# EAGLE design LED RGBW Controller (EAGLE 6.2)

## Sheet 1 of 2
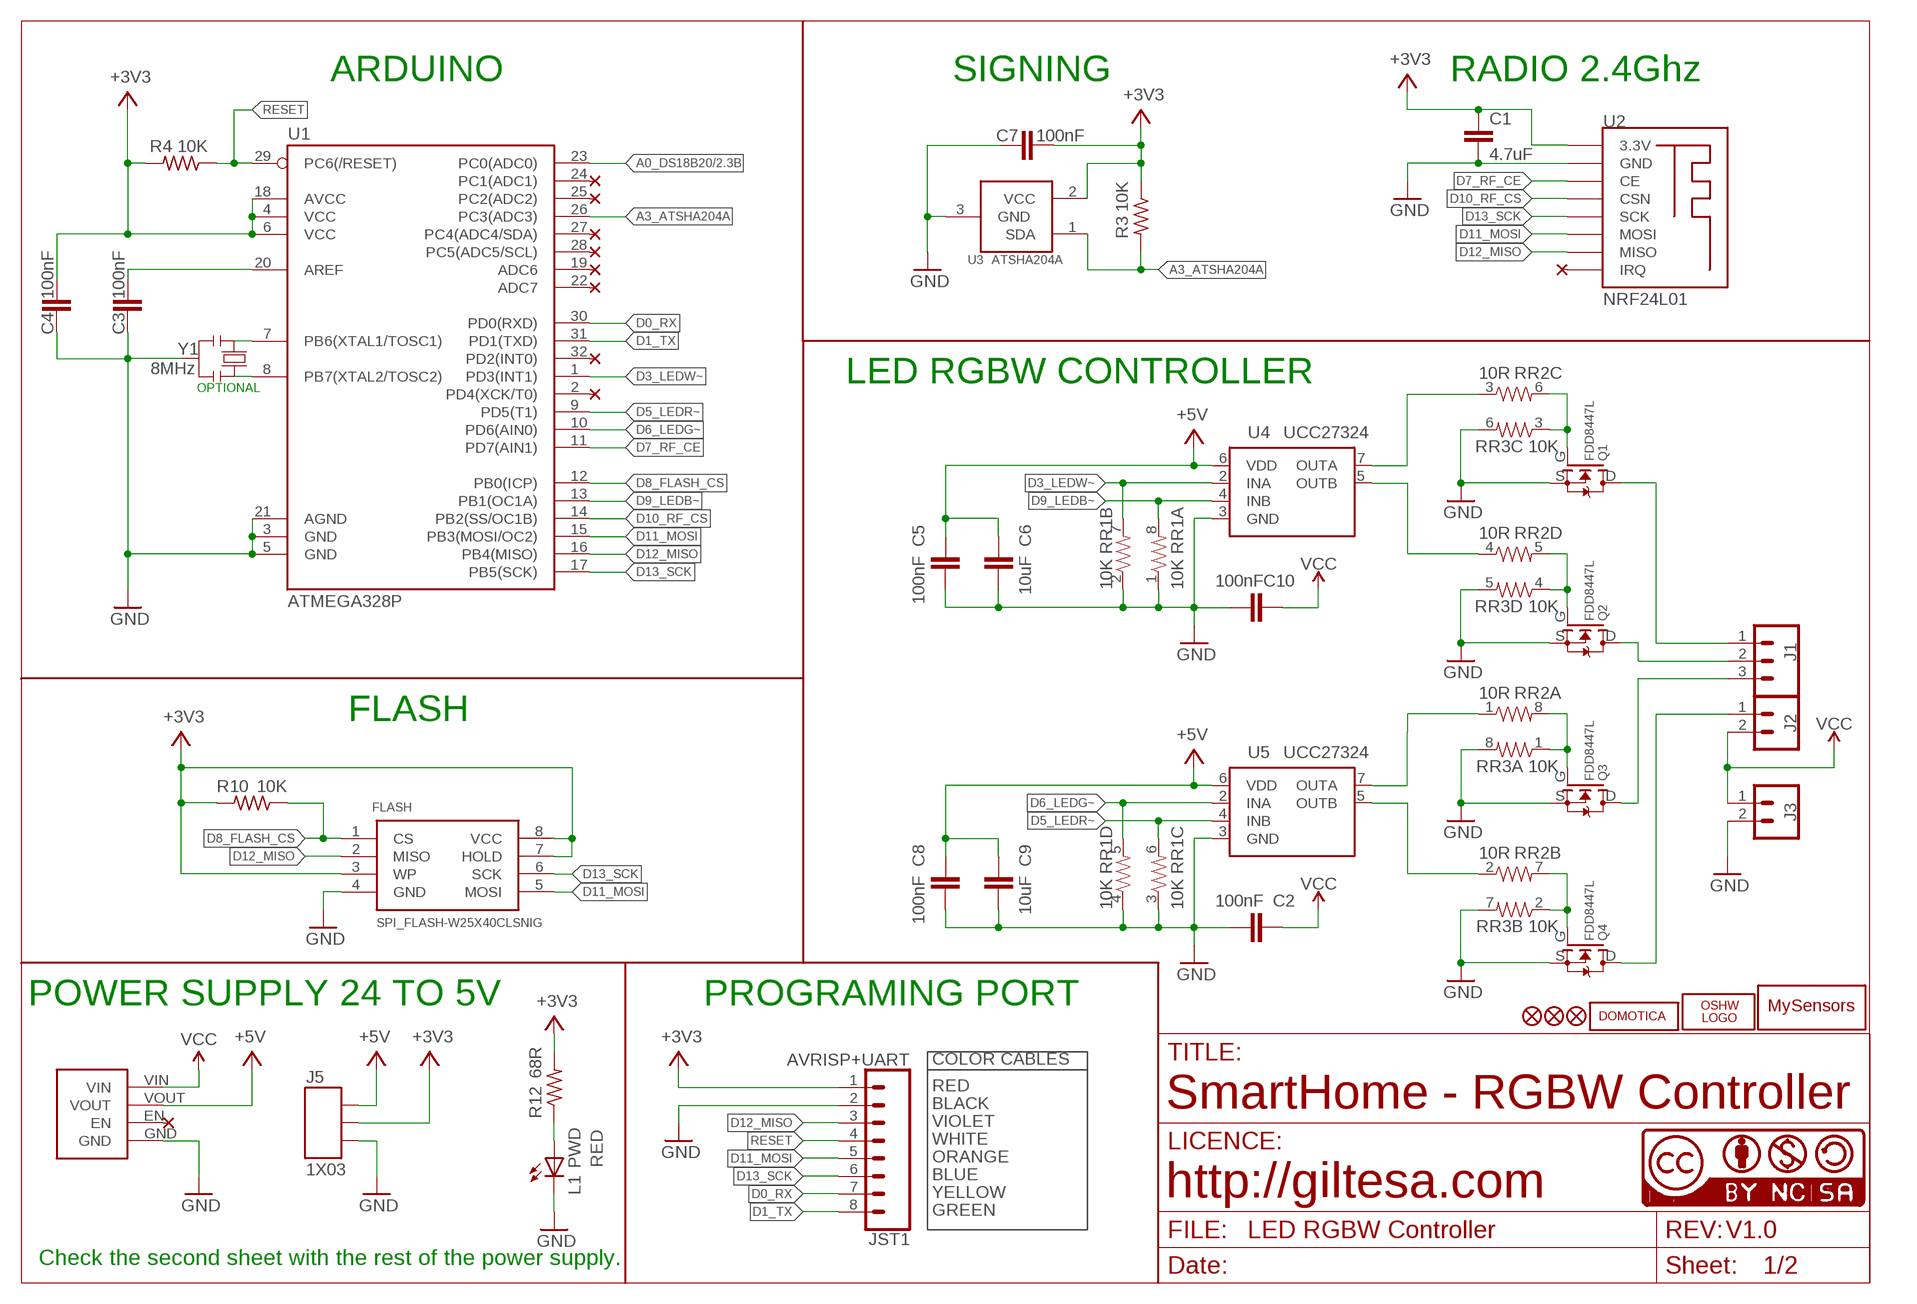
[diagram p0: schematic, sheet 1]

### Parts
C1  4.7uF  C1206  [C1206]
C2  100nF  C0603  [C0603]
C3  100nF  C0603  [C0603]
C4  100nF  C0603  [C0603]
C5  100nF  C0603  [C0603]
C6  10uF  C0603  [C0603]
C7  100nF  C0603  [C0603]
C8  100nF  C0603  [C0603]
C9  10uF  C0603  [C0603]
C10  100nF  C0603  [C0603]
FLASH  SPI_FLASH-W25X40CLSNIG  SPI_FLASH-X25XXSMD  [SO08]
J1  TERMINAL_5MM_3P  [TERMINAL_5MM_3P]
J2  TERMINAL_5MM_2P1  [TERMINAL_5MM_2P]
J3  TERMINAL_5MM_2P1  [TERMINAL_5MM_2P]
J4  DC_CONVERTER  [DC_CONVERTER]
J5  1X03  [1X03_SMD]
JST1  AVRISP+UART  JST-8-1MM-SMD1  [JST-8-1MM-SMD]
L1  PWD  LEDCHIP-LED0805  [CHIP-LED0805]
LOGO1  OSHW_LOGO_FILLX0150-NT  [OSHW_FILLX150_NOTEXT]
Q1  FDD8447L  [TO-252]
Q2  FDD8447L  [TO-252]
Q3  FDD8447L  [TO-252]
Q4  FDD8447L  [TO-252]
R3  10K  R0603  [R0603]
R4  10K  R0603  [R0603]
R10  10K  R0603  [R0603]
R12  68R  R0603  [R0603]
RR1  10K  RESISTOR-ARRAY0603-ARV  [0603-ARV]
RR2  10R  RESISTOR-ARRAY0603-ARV  [0603-ARV]
RR3  10K  RESISTOR-ARRAY0603-ARV  [0603-ARV]
U1  ATMEGA328P  ATMEGA328P_TQFP  [TQFP32-08]
U2  NRF24L01  NRF24L01_SMD  [NRF24L01_SMD]
U3  ATSHA204A  IC_ATSHA204A_CRYPT  [SOT23-3]
U4  UCC27324  [SO8]
U5  UCC27324  [SO8]
U$2  MYSENSORS3  [MYSENSORS_15MM]
U$5  DOMOTICA10MM_2  [DOMOTICA-10MM_2]
U$6  FIDUCIAL1X2  [FIDUCIAL-1X2]
U$7  FIDUCIAL1X2  [FIDUCIAL-1X2]
U$12  CC-BY-NC-SA15MM  [CC-BY-NC-SA_15MM]
U$14  FIDUCIAL1X2  [FIDUCIAL-1X2]
U$18  CC-NC-BCNIX  [CC-NC-B_NIX]
Y1  8MHz  RESONATORMU  [RESONATOR]

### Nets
+3V3: C1.1 C4.2 C7.2 FLASH.3(WP) FLASH.7(HOLD) FLASH.8(VCC) J5.2 JST1.1 R3.1 R4.2 R10.2 R12.2 U1.4(VCC) U1.6(VCC) U1.18(AVCC) U2.3.3V U3.2(VCC) ; also sheet 2
+5V: C5.2 C6.2 C8.2 C9.2 J4.VOUT J5.3 U4.6(VDD) U5.6(VDD)
A0_DS18B20: U1.23(PC0(ADC0)) ; also sheet 2
A3_ATSHA204A: R3.2 U1.26(PC3(ADC3)) U3.1(SDA)
D0_RX: JST1.7 U1.30(PD0(RXD))
D1_TX: JST1.8 U1.31(PD1(TXD))
D3_LEDW~: RR1.7 U1.1(PD3(INT1)) U4.2(INA)
D5_LEDR~: RR1.6 U1.9(PD5(T1)) U5.4(INB)
D6_LEDG~: RR1.5 U1.10(PD6(AIN0)) U5.2(INA)
D7_RF_CE: U1.11(PD7(AIN1)) U2.CE
D8_FLASH_CS: FLASH.1(CS) R10.1 U1.12(PB0(ICP))
D9_LEDB~: RR1.8 U1.13(PB1(OC1A)) U4.4(INB)
D10_RF_CS: U1.14(PB2(SS/OC1B)) U2.CSN
D11_MOSI: FLASH.5(MOSI) JST1.5 U1.15(PB3(MOSI/OC2)) U2.MOSI
D12_MISO: FLASH.2(MISO) JST1.3 U1.16(PB4(MISO)) U2.MISO
D13_SCK: FLASH.6(SCK) JST1.6 U1.17(PB5(SCK)) U2.SCK
GND: C1.2 C2.1 C3.1 C4.1 C5.1 C6.1 C7.1 C8.1 C9.1 C10.1 FLASH.4(GND) J3.2 J4.GND J5.1 JST1.2 L1.C Q1.S Q2.S Q3.S Q4.S RR1.1 RR1.2 RR1.3 RR1.4 RR3.5 RR3.6 RR3.7 RR3.8 U1.3(GND) U1.5(GND) U1.21(AGND) U2.GND U3.3(GND) U4.3(GND) U5.3(GND) Y1.2 ; also sheet 2
N$1: J1.1 Q1.D
N$2: Q2.G RR2.5 RR3.4
N$3: J1.2 Q2.D
N$4: Q3.G RR2.8 RR3.1
N$5: J1.3 Q3.D
N$6: Q1.G RR2.6 RR3.3
N$7: Q4.G RR2.7 RR3.2
N$8: J2.1 Q4.D
N$9: L1.A R12.1
N$10: RR2.3 U4.7(OUTA)
N$11: RR2.4 U4.5(OUTB)
N$12: RR2.1 U5.7(OUTA)
N$13: RR2.2 U5.5(OUTB)
N$29: U1.7(PB6(XTAL1/TOSC1)) Y1.1
N$30: U1.8(PB7(XTAL2/TOSC2)) Y1.3
N$33: C3.2 U1.20(AREF)
RESET: JST1.4 R4.1 U1.29(PC6(/RESET))
VCC: C2.2 C10.2 J2.2 J3.1 J4.VIN
Unconnected: J4.EN U1.2(PD4(XCK/T0)) U1.19(ADC6) U1.22(ADC7) U1.24(PC1(ADC1)) U1.25(PC2(ADC2)) U1.27(PC4(ADC4/SDA)) U1.28(PC5(ADC5/SCL)) U1.32(PD2(INT0)) U2.IRQ

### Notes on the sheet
- ARDUINO | SIGNING | RADIO 2.4Ghz
- LED RGBW CONTROLLER
- OPTIONAL
- FLASH
- POWER SUPPLY 24 TO 5V | PROGRAMING PORT
- COLOR CABLES
- RED
- BLACK | SmartHome - RGBW Controller
- VIOLET
- WHITE
- RED | ORANGE
- BLUE
- YELLOW | http://giltesa.com
- GREEN
- V1.0
- Check the second sheet with the rest of the power supply.

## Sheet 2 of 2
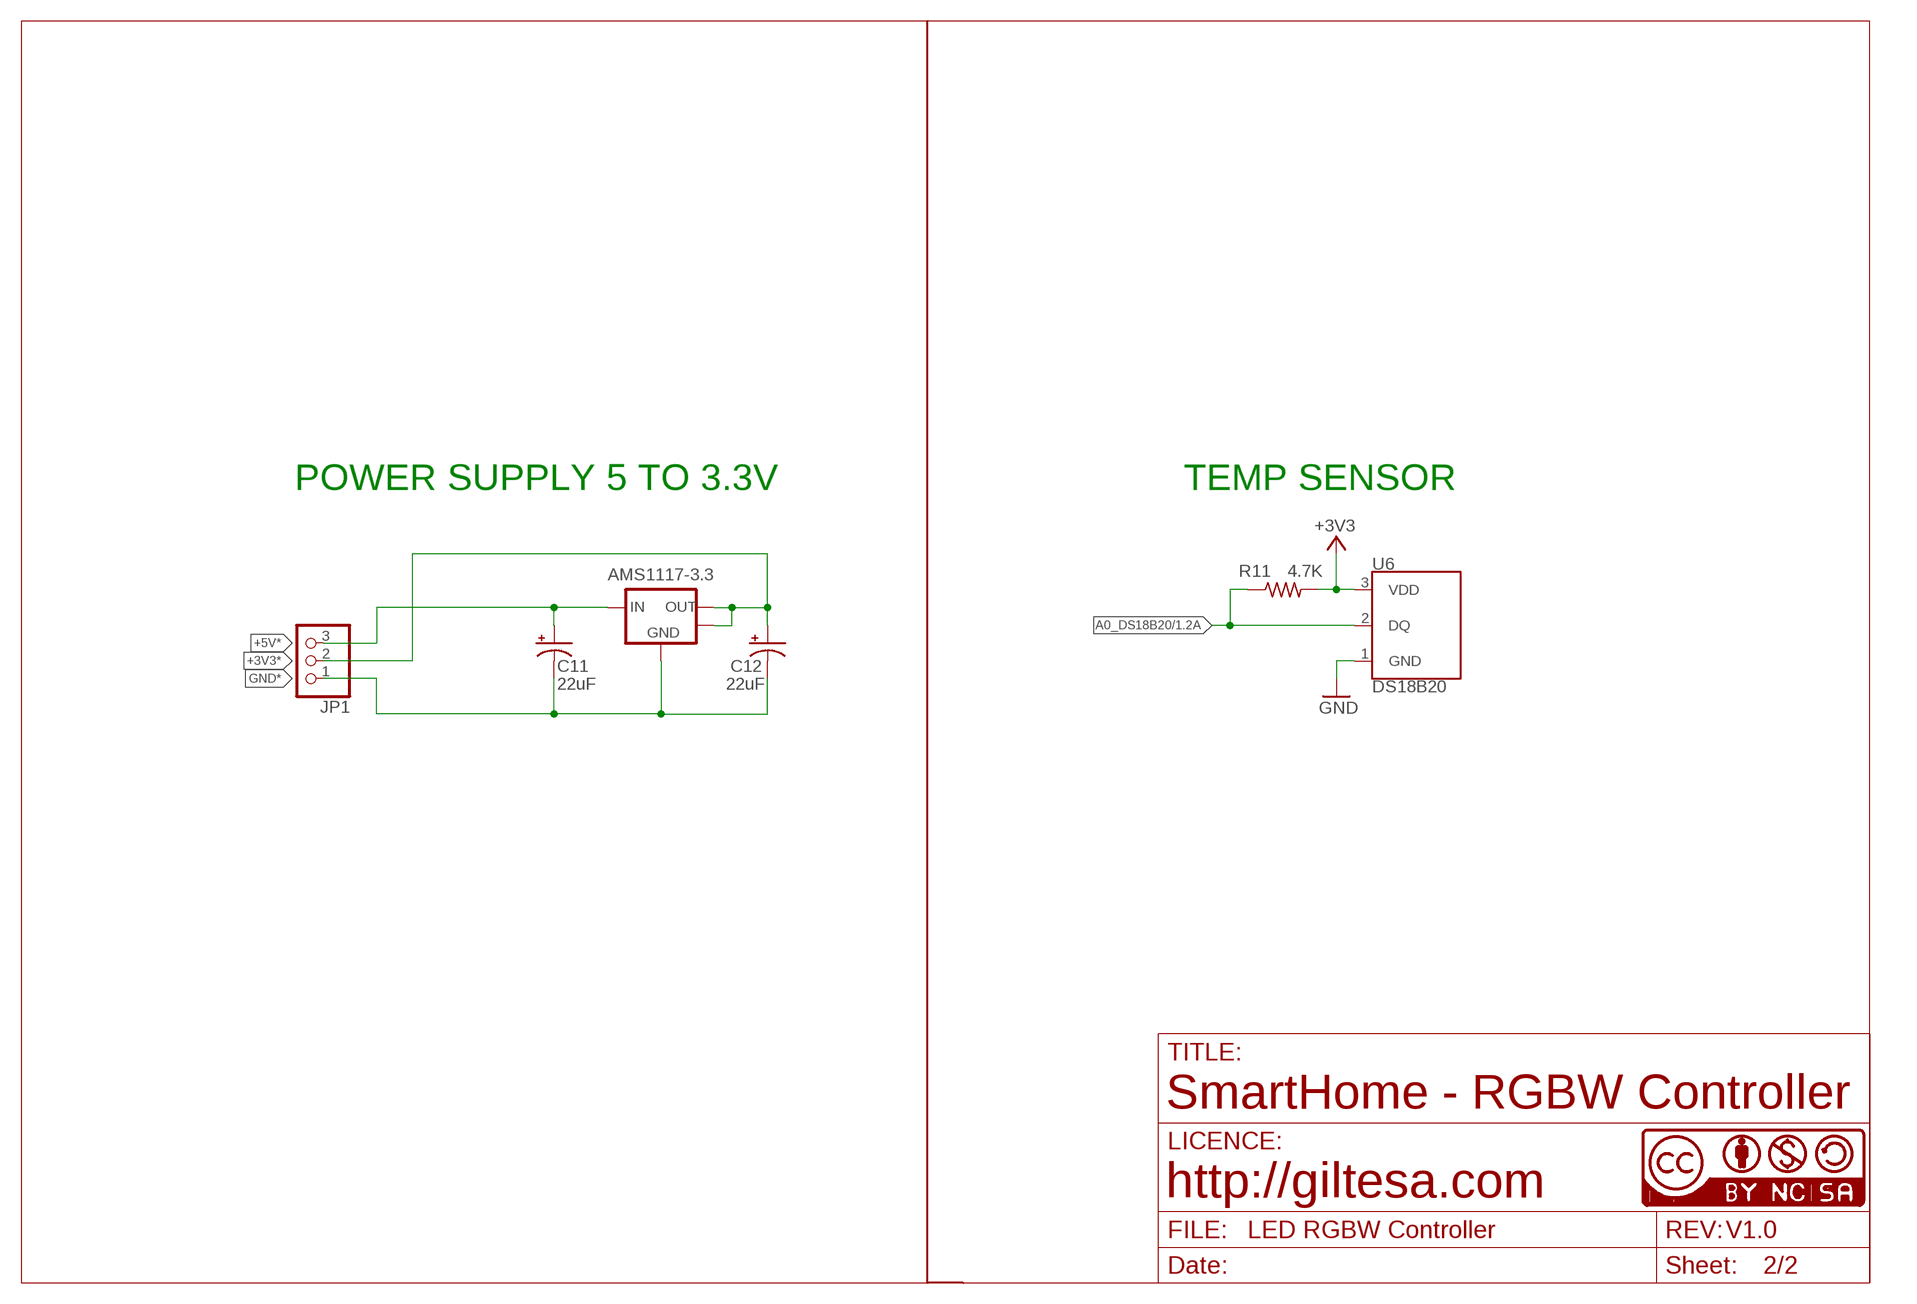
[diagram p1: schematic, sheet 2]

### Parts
AMS1117-3.3  AMS1117-3.3  AMS1117SOT89_2  [SOT89_2]
C11  22uF  CAP_POL3528  [EIA3528]
C12  22uF  CAP_POL3528  [EIA3528]
JP1  PINHD-1X3  [1X03]
R11  4.7K  R0603  [R0603]
U6  DS18B20  [DS18B20]
U$21  CC-NC-BCNIX  [CC-NC-B_NIX]

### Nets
+3V3: R11.2 U6.3(VDD) ; also sheet 1
+3V3*: AMS1117-3.3.2(OUT) AMS1117-3.3.4(NC) C12.A(+) JP1.2
+5V*: AMS1117-3.3.3(IN) C11.A(+) JP1.3
A0_DS18B20: R11.1 U6.2(DQ) ; also sheet 1
GND: U6.1(GND) ; also sheet 1
GND*: AMS1117-3.3.1(GND) C11.C(-) C12.C(-) JP1.1

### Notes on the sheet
- POWER SUPPLY 5 TO 3.3V | TEMP SENSOR
- SmartHome - RGBW Controller
- http://giltesa.com
- V1.0

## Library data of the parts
AMS1117-3.3 = ,giltesa:AMS1117
C1 = ,giltesa:C1206
C2-C10 = ,giltesa:C0603
C11 C12 = SparkFun:CAP_POL: Capacitor Polarized
FLASH = SparkFun-DigitalIC:SPI_FLASH-X25XX: 8pin SPI Flash series x25xx. Works with devices like W25X32 and BR25L32
J1 = ,giltesa:TERMINAL_5MM_3P
J2 J3 = ,giltesa:TERMINAL_5MM_2P
J4 = ,giltesa:DC_CONVERTER
J5 = ,giltesa:1X03
JP1 = adafruit:PINHD-1X3: PIN HEADER
JST1 = ,giltesa:JST-8-1MM-SMD
L1 = led:LED: LED
LOGO1 = ohw-logo:OSHW_LOGO_FILL
Q1-Q4 = ,giltesa:FDD8447L
R3 R4 R10-R12 = ,giltesa:R0603
RR1-RR3 = SparkFun-Passives:RESISTOR-ARRAY: Array Chip Resistor Source: RS Component / Phycomp
U1 = SparkFun-DigitalIC:ATMEGA328P_TQFP; PROD_ID: IC-09069; VALUE: ATMEGA328P_TQFP
U2 = ,giltesa:NRF24L01_SMD
U3 = TD-MySensors:IC_ATSHA204A_CRYPT
U4 U5 = ,giltesa:UCC27324
U6 = ,giltesa:DS18B20
U$2 = ,giltesa_logos:MYSENSORS
U$5 = ,giltesa_logos:DOMOTICA
U$6 U$7 U$14 = SparkFun:FIDUCIAL: Fiducial Alignment Points
U$12 = ,giltesa_logos:CC-BY-NC-SA
U$18 U$21 = cc-by-nc-sa:CC-NC-BC: All hardware is licensed under the Creative Commons
Y1 = MySMD2:RESONATOR

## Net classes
2 gnd: width 0.305 mm, drill 0.406 mm, clearance 0.203 mm
3 usbvcc: width 0.203 mm, drill 0.406 mm, clearance 0.203 mm
4 USBpair: width 0.254 mm, drill 0.406 mm, clearance 0.61 mm

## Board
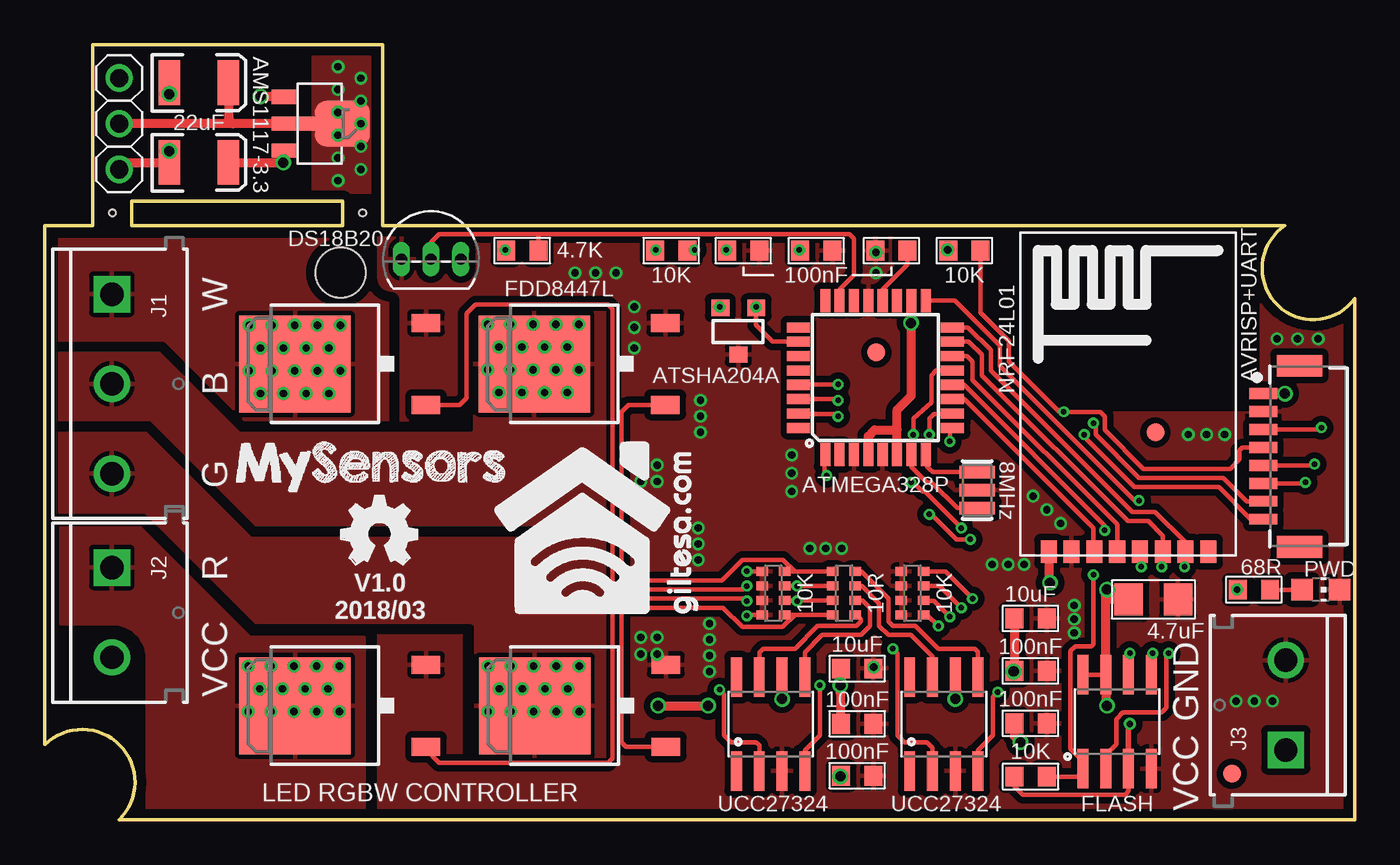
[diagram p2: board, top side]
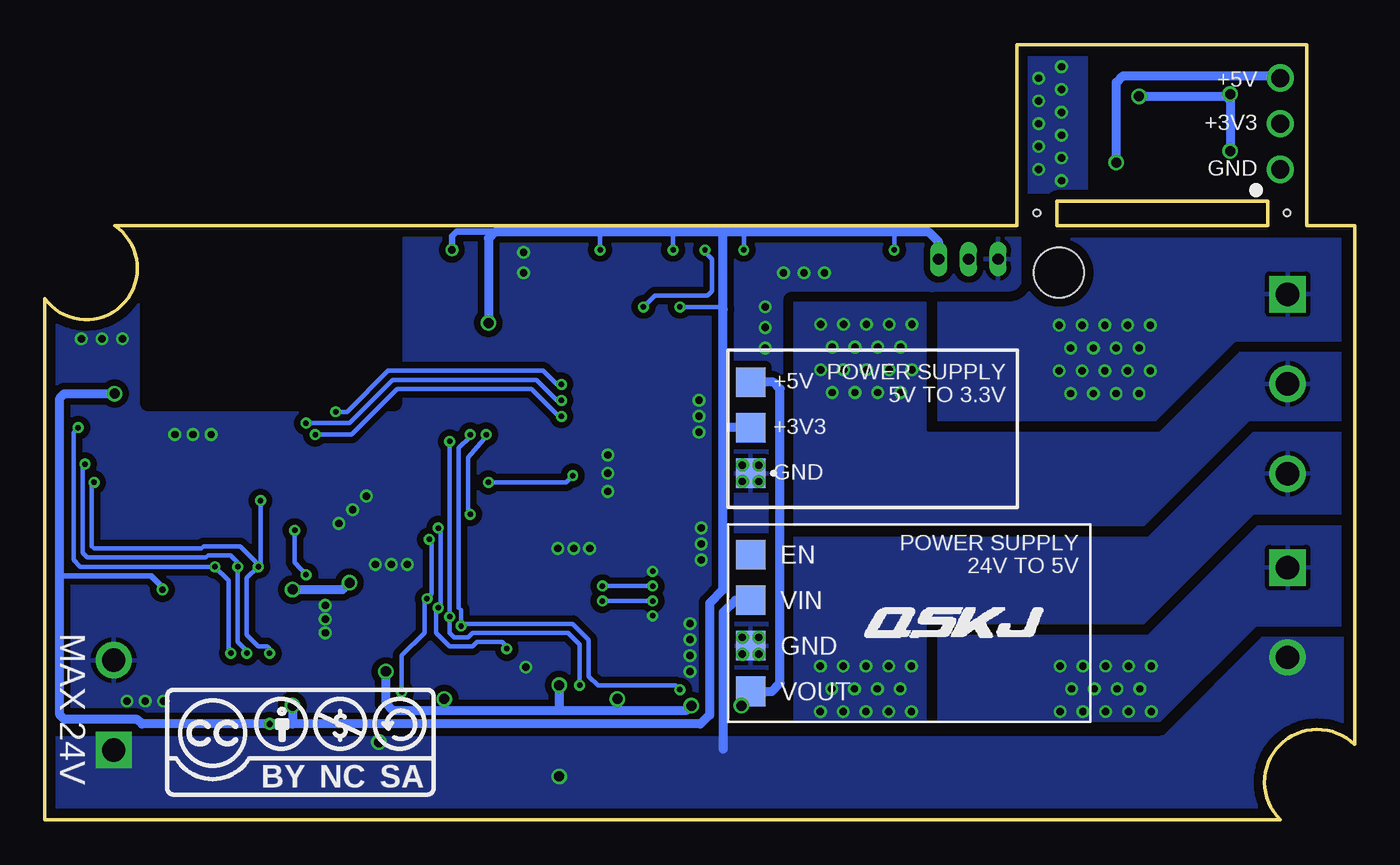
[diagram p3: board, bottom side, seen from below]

Size 72.97 x 43.18 mm. Coordinates in mm from the lower left corner, seen from the top.
Outline: 4.14,0 72.97,0 72.97,29.03 arc-200 69.09,33.1 18.82,33.1 18.82,43.18 2.67,43.18 2.67,33.1 0,33.1 0,4.19 0.03,4.19 arc-180 4.14,0
Outline: 16.59,33.1 4.85,33.1 4.85,34.47 16.59,34.47 16.59,33.1
Copper layers (1*16): Top 0.035mm / dielectric 1.6mm / Bottom 0.035mm
Design rules: minimum track width 6mil, minimum drill 12mil, track to track 6mil, track to pad 6mil, pad to pad 6mil, via to via 8mil, smd to smd 0mil, copper to edge 20mil, drill to drill 10mil, minimum pad ring 6mil, minimum via ring 6mil, stop-mask expansion 0mil, vias tented up to drill 100mil, thermal gap 10mil
Holes 0.38 mm at 17.7,33.81 3.76,33.81
Holes 2.79 mm at 16.47,30.49
tRestrict: 41 lines
bRestrict: 44 lines

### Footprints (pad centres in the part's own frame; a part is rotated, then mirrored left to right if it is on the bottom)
SOT89_2 = smd 0.8 x 1.4: 1 -1.499,-1.981; 3 1.499,-1.981 | smd 0.8 x 2.54: 2 0,-1.409 | smd 2.54 x 3.048: 4 0,1.27
C1206 = smd 1.6 x 1.8: 1 -1.362,-0.013; 2 1.387,-0.013
C0603 = smd 1 x 1.1: 1 -0.901,-0.038; 2 0.901,-0.038
EIA3528 = smd 1.2 x 2.5: A 1.65,0; C -1.65,0
SO08 = smd 0.61 x 2.21: 1 -1.905,-2.616; 2 -0.635,-2.616; 3 0.635,-2.616; 4 1.905,-2.616; 5 1.905,2.616; 6 0.635,2.616; 7 -0.635,2.616; 8 -1.905,2.616
TERMINAL_5MM_3P = drill 1.3 pad 2.032 square: 1 0,0 | drill 1.3 pad 2.032: 2 5,0; 3 10,0
TERMINAL_5MM_2P = drill 1.3 pad 2.032 square: 1 0,0 | drill 1.3 pad 2.032: 2 5,0
DC_CONVERTER = smd 1.651 x 1.651: EN 1.27,9.31; GND 1.27,4.23; VIN 1.27,6.77; VOUT 1.27,1.69
1X03_SMD = smd 1.651 x 1.651: 1 0,-2.54; 2 0,0; 3 0,2.54
1X03 = drill 1.016: 1 -2.54,0; 2 0,0; 3 2.54,0
JST-8-1MM-SMD = smd 0.6 x 1.55: 1 -3.5,-2.017; 2 -2.5,-2.017; 3 -1.5,-2.017; 4 -0.5,-2.017; 5 0.5,-2.017; 6 1.5,-2.017; 7 2.5,-2.017; 8 3.5,-2.017 | smd 1.219 x 2.54: NC1 -5.054,0; NC2 5.054,0
CHIP-LED0805 = smd 1.2 x 1.2: A 0,-1.05; C 0,1.05
TO-252 = smd 5.4 x 6.2: D 0,2.5 | smd 1 x 1.6: G -2.28,-4.8; S 2.28,-4.8
R0603 = smd 1 x 1.1: 1 -0.901,0.013; 2 0.901,0.013
0603-ARV = smd 0.5 x 0.65: 1 -1.2,-0.625; 2 -0.4,-0.625; 3 0.4,-0.625; 4 1.2,-0.625; 5 1.2,0.625; 6 0.4,0.625; 7 -0.4,0.625; 8 -1.2,0.625
TQFP32-08 = smd 1.27 x 0.559: 1 -4.293,2.8; 2 -4.293,2; 3 -4.293,1.2; 4 -4.293,0.4; 5 -4.293,-0.4; 6 -4.293,-1.2; 7 -4.293,-2; 8 -4.293,-2.8; 17 4.293,-2.8; 18 4.293,-2; 19 4.293,-1.2; 20 4.293,-0.4; 21 4.293,0.4; 22 4.293,1.2; 23 4.293,2; 24 4.293,2.8 | smd 0.559 x 1.27: 9 -2.8,-4.293; 10 -2,-4.293; 11 -1.2,-4.293; 12 -0.4,-4.293; 13 0.4,-4.293; 14 1.2,-4.293; 15 2,-4.293; 16 2.8,-4.293; 25 2.8,4.293; 26 2,4.293; 27 1.2,4.293; 28 0.4,4.293; 29 -0.4,4.293; 30 -1.2,4.293; 31 -2,4.293; 32 -2.8,4.293
NRF24L01_SMD = smd 0.9 x 1.27: 3.3V 1.575,0.203; CE 4.115,0.203; CSN 5.385,0.203; GND 2.845,0.203; IRQ 10.465,0.203; MISO 9.195,0.203; MOSI 7.925,0.203; SCK 6.655,0.203
SOT23-3 = smd 1 x 0.9: 1 -1,-1.3; 2 1,-1.3; 3 0,1.3
SO8 = smd 0.61 x 2.21: 1 -1.905,-2.616; 2 -0.635,-2.616; 3 0.635,-2.616; 4 1.905,-2.616; 5 1.905,2.616; 6 0.635,2.616; 7 -0.635,2.616; 8 -1.905,2.616
DS18B20 = drill 0.635 pad 0.864 long: 1 -1.651,0; 2 0,0; 3 1.651,0
FIDUCIAL-1X2 = smd 1 x 1: 1 0,0
RESONATOR = smd 0.7 x 2: 1 -1,0; 2 0,0; 3 1,0

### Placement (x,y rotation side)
AMS1117-3.3  15.32,38.79 270 top
C1  61.75,12.29 0 top
C2  45.26,2.41 180 top
C3  47.17,31.75 0 top
C4  42.98,31.67 180 top
C5  54.91,8.26 180 top
C6  54.91,11.18 180 top
C7  38.91,31.67 180 top
C8  45.26,5.31 180 top
C9  45.26,8.38 180 top
C10  54.91,5.33 180 top
C11  8.59,36.63 0 top
C12  8.59,41.07 0 top
FLASH  59.74,5.46 0 top
J1  3.73,29.29 270 top
J2  3.73,14.05 270 top
J3  69.14,3.89 90 top
J4  34.92,5.46 0 bottom
J5  33.66,21.84 0 bottom
JP1  4.14,38.79 90 top
JST1  69.9,20.24 270 top
L1  71.09,12.83 270 top
LOGO1  16.51,14.22 0 top
Q1  16.43,25.4 90 top
Q2  29.77,25.4 90 top
Q3  29.79,6.35 90 top
Q4  16.43,6.35 90 top
R3  34.9,31.7 0 top
R4  51.23,31.72 180 top
R10  54.91,2.41 180 top
R11  26.59,31.72 180 top
R12  67.36,12.83 180 top
RR1  48.34,12.62 270 top
RR2  44.53,12.62 90 top
RR3  40.59,12.62 90 top
U1  46.28,24.64 90 top
U2  54.36,14.73 0 top
U3  38.63,27.23 180 top
U4  50.09,5.33 0 top
U5  40.44,5.33 0 top
U6  21.51,31.24 0 top
U$2  10.67,18.29 0 top
U$5  25.65,11.3 0 top
U$6  46.33,26.04 180 top
U$7  61.87,21.59 180 top
U$12  66.29,1.27 0 bottom
U$14  66.14,2.57 180 top
U$18  0,0 180 top
U$21  0,0 180 top
Y1  51.94,18.36 90 top

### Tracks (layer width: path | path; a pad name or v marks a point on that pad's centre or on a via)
+3V3  (via drill 0.3, 0.36, 0.41, 0.56)
  Top 0.254: C4.2 42.08,32.09 v42.04,31.75 | R11.2 25.69,31.96 v25.65,31.75 | C7.2 38.01,31.96 v37.97,31.75 | U3.2 37.38,28.53 v37.59,28.57 | FLASH.8 FLASH.7 | v34.04,31.75 34.01,31.75 R3.1 | R10.2 54.01,1.87 54.48,1.4 60.2,1.4 60.38,1.57 FLASH.3
  Top 0.305: FLASH.3 60.38,5.26 v60.45,5.33 | R12.2 66.53,12.81 v66.42,12.83
  Top 0.356: R4.2 50.33,31.96 v50.29,31.75
  Top 0.508: v69.09,23.75 JST1.1 | v59.18,6.35 59.11,6.43 FLASH.7 59.11,12.32 | 59.11,12.32 59.11,12.88 v59.18,12.83 | 56.01,13.08 v56.01,13.21 55.93,13.28 U2.3.3V | C1.1 59.14,12.28 59.11,12.32 | U1.6 47.48,21.72 | 47.48,21.72 47.48,22.84 48.26,23.62 v48.26,27.69 48.26,28.91 U1.18 | U1.4 45.88,21.37 46.23,21.72 47.48,21.72
  Bottom 0.254: 35.81,32.64 35.69,32.77 | v42.04,31.75 42.04,32.64 41.91,32.77 | v25.65,31.75 25.65,32.77 | v37.97,31.75 37.97,32.64 38.1,32.77 | v37.59,28.57 35.31,28.57 35.18,28.45 | v34.04,31.75 34.04,32.64 34.16,32.77
  Bottom 0.305: v60.45,5.33 60.2,5.33 | v66.42,12.83 66.42,12.95 67.06,13.59 72.14,13.59
  Bottom 0.356: v50.29,31.75 50.29,32.51 50.04,32.77 47.75,32.77
  Bottom 0.508: 59.18,5.33 36.45,5.33 35.94,5.84 35.94,12.06 35.18,12.83 35.18,21.72 | 59.18,5.33 60.2,5.33 67.56,5.33 67.82,5.59 71.88,5.59 72.14,5.84 72.14,13.59 72.14,23.5 71.88,23.75 v69.09,23.75 | 35.18,21.72 35.18,28.45 35.18,32.77 | 35.18,32.77 35.69,32.77 38.1,32.77 41.91,32.77 47.75,32.77 47.88,32.77 48.26,32.38 v48.26,27.69 | 35.18,32.77 34.16,32.77 25.65,32.77 23.75,32.77 23.16,32.18 U6.3 | J5.2 35.05,21.84 35.18,21.72 | v59.18,6.35 59.18,5.33 | v59.18,12.83 56.39,12.83 v56.01,13.21
+3V3*  (via drill 0.41)
  Top 0.508: AMS1117-3.3.4 AMS1117-3.3.2 10.49,38.79 | 10.49,38.79 JP1.2 | C12.A 10.23,39.04 10.49,38.79
  other vias: 17.6,38.79 17.6,40.06 17.6,41.33 17.6,37.52 17.6,36.25 16.33,36.88 16.33,38.15 16.33,39.42 16.33,40.69 16.33,41.96 16.33,35.61
  pour Top (no thermals): 14.94,42.72 18.49,42.72 18.49,34.98 14.94,34.98
  pour Bottom (no thermals): 14.94,42.72 18.49,42.72 18.49,34.98 14.94,34.98
+5V  (via drill 0.56)
  Top 0.508: v34.16,6.35 v36.96,6.35 | v53.98,8.26 v53.98,8.25 C5.2 C6.2 | U4.6 v50.72,6.73 | U5.6 v41.07,6.73 | C8.2 44.36,7.28 | 44.36,6.44 v44.32,7.49 44.36,7.28 | C9.2 44.36,7.28
  Bottom 0.508: J5.3 32.38,24.38 32,24 32,7.62 32.47,7.15 J4.VOUT v34.16,6.35 | v53.98,8.26 53.98,6.48 53.59,6.1 50.85,6.1 | 50.85,6.1 44.45,6.1 | 44.45,6.1 41.07,6.1 | 41.07,6.1 37.21,6.1 v36.96,6.35 | v41.07,6.73 41.07,6.1 | v50.72,6.73 50.72,6.22 50.85,6.1 | v44.32,7.49 44.32,6.22 44.45,6.1
+5V*  (via drill 0.56)
  Top 0.508: AMS1117-3.3.3 13.34,36.68 v13.28,36.63 C11.A
  Bottom 0.508: v13.28,36.63 13.28,41.07 12.9,41.45 4.27,41.45 JP1.3
A0_DS18B20
  Top 0.254: U1.23 44.28,29.55 45.09,30.35 45.09,32.38 44.83,32.64 27.43,32.64 | 27.43,32.64 21.97,32.64 21.51,32.18 U6.2 | R11.1 27.5,32.58 27.43,32.64
A3_ATSHA204A  (via drill 0.3)
  Top 0.254: R3.2 36.16,31.71 v36.2,31.75 | U1.26 40.55,26.64 39.62,27.56 39.62,28.52 | 39.62,28.52 U3.1 39.71,28.45 v39.62,28.57 39.62,28.52
  Bottom 0.254: v36.2,31.75 36.2,31.62 35.81,31.24 35.81,29.46 36.07,29.21 38.99,29.21 v39.62,28.57 39.5,28.7
D0_RX  (via drill 0.3)
  Top 0.254: JST1.7 66.97,17.74 65.66,19.05 60.96,19.05 58.55,21.46 58.55,21.97 v58.42,22.1 | U1.30 44.13,23.44 v44.2,23.37
  Bottom 0.254: v44.2,23.37 44.45,23.37 45.59,24.51 53.59,24.51 56.01,22.1 v58.42,22.1
D1_TX  (via drill 0.3)
  Top 0.254: JST1.8 67.2,16.74 65.41,18.54 60.71,18.54 57.91,21.34 v57.91,21.46 | U1.31 42.02,22.61 44.07,22.61 v44.2,22.48
  Bottom 0.254: v44.2,22.48 44.32,22.48 45.85,24 53.34,24 55.88,21.46 v57.91,21.46
D3_LEDW~  (via drill 0.3)
  Top 0.254: U4.2 49.45,4.01 49.15,4.32 47.88,4.32 47.5,4.7 47.5,9.27 v47.24,9.53 | RR1.7 49.84,13.02 v51.05,11.81 | v51.05,16.26 49.02,18.29 48.9,18.29 48.39,18.8 v48.26,18.8 | U1.1 43.43,20.3 43.43,19.3 v43.56,19.18
  Bottom 0.254: v47.24,9.53 47.24,9.65 47.5,9.91 48.9,9.91 49.15,9.65 50.42,9.65 51.18,10.41 51.18,11.68 v51.05,11.81 50.93,11.94 50.93,16.13 v51.05,16.26 | v48.26,18.8 43.94,18.8 v43.56,19.18
D5_LEDR~  (via drill 0.3)
  Top 0.254: RR1.6 48.99,12.19 49.53,12.19 v50.42,11.3 | v43.18,7.49 43.18,4.7 42.34,3.86 U5.4 | v50.42,21.08 50.42,21.69 U1.9
  Bottom 0.254: v43.18,7.49 43.18,9.78 43.81,10.41 49.15,10.41 49.4,10.16 50.16,10.16 50.42,10.41 v50.42,11.3 v50.42,21.08
D6_LEDG~  (via drill 0.3)
  Top 0.254: U5.2 39.8,4.14 39.62,4.32 38.23,4.32 37.85,4.7 37.85,6.99 v37.59,7.24 | RR1.5 49.16,11.42 v49.78,10.79 | v49.28,21.46 49.28,22.35 49.53,22.61 50.54,22.61 U1.10
  Bottom 0.254: v37.59,7.24 37.85,7.49 42.16,7.49 42.67,8 42.67,10.03 43.56,10.92 49.66,10.92 v49.78,10.79 49.78,11.68 49.91,11.81 49.91,20.7 49.28,21.34 v49.28,21.46
D7_RF_CE
  Top 0.254: U2.CE 58.47,15.19 58.42,15.24 58.42,16.26 51.24,23.44 U1.11
D8_FLASH_CS  (via drill 0.3)
  Top 0.254: v58.42,13.65 58.42,9.78 58.29,9.65 57.4,9.65 57.15,9.4 57.15,3.94 57.84,3.25 FLASH.1 57.84,2.41 57.53,2.41 57.52,2.4 R10.1 | U1.12 51.2,24.24 59.05,16.38 v59.05,16.13
  Bottom 0.254: v58.42,13.65 59.05,14.35 v59.05,16.13
D9_LEDB~  (via drill 0.3)
  Top 0.254: U4.4 51.99,3.86 52.83,4.7 52.83,6.86 v53.09,7.11 | RR1.8 48.98,13.84 50.16,13.84 v51.69,12.32 | U1.13 50.55,25.02 49.66,25.02 49.4,24.77 49.4,23.24 48.39,22.35 v48.39,21.46 | v51.56,15.62 50.8,15.62 49.4,17.02 v49.28,17.02
  Bottom 0.254: v53.09,7.11 53.09,9.14 51.82,10.41 51.82,12.19 v51.69,12.32 51.44,12.57 51.44,15.49 v51.56,15.62 | v49.28,17.02 49.4,17.02 49.4,20.19 48.51,21.21 v48.39,21.46
D10_RF_CS
  Top 0.254: U2.CSN 59.74,16.46 51.69,24.51 51.69,25.53 51.38,25.84 U1.14
D11_MOSI  (via drill 0.3)
  Top 0.254: v62.23,14.1 62.28,14.15 U2.MOSI 62.28,15.82 61.47,16.64 60.33,16.64 52.2,24.77 52.2,25.91 51.47,26.64 U1.15 | v61.72,9.27 61.72,8.15 FLASH.5 | JST1.5 70.67,19.74 v70.74,19.81
  Bottom 0.254: v61.72,9.27 61.72,9.4 62.23,9.91 v62.23,14.1 62.23,14.35 62.61,14.73 63.88,14.73 64.01,14.61 70.61,14.61 70.87,14.86 70.87,19.68 v70.74,19.81
D12_MISO  (via drill 0.3)
  Top 0.254: v62.61,9.27 62.48,9.14 62.48,6.22 62.23,5.97 60.07,5.97 59.69,5.59 59.69,4.19 59.11,3.61 FLASH.2 | v63.5,14.1 63.5,14.76 U2.MISO 63.5,14.99 63.5,15.49 61.85,17.14 60.58,17.14 52.7,25.02 52.7,26.16 51.43,27.44 U1.16 | JST1.3 71.02,21.74 v71.12,21.84
  Bottom 0.254: v62.61,9.27 62.74,9.4 62.74,13.34 v63.5,14.1 70.99,14.1 71.37,14.48 71.37,21.59 v71.12,21.84
D13_SCK  (via drill 0.3)
  Top 0.254: U2.SCK 61.01,14.17 v61.09,14.1 | v60.45,9.27 60.45,8.15 FLASH.6 | JST1.6 70.18,18.74 v70.23,18.8 | U1.17 50.7,28.93 53.21,26.42 53.21,25.27 60.83,17.65 v60.96,17.78
  Bottom 0.254: v60.45,9.27 60.45,9.53 60.58,9.65 61.09,9.65 61.72,10.29 61.72,13.46 v61.09,14.1 | v61.09,14.1 61.09,14.22 62.1,15.24 64.14,15.24 64.26,15.11 70.23,15.11 70.36,15.24 70.36,18.67 v70.23,18.8 | v60.96,17.78 60.96,14.22 v61.09,14.1
GND  (via drill 0.3, 0.41)
  Top 0.254: RR3.5 39.13,13.82 v39.12,13.84 | RR3.8 39.12,11.42 v39.12,11.37
  other vias: 33.2,10.16 34.11,10.16 33.2,9.22 34.11,9.22 33.2,18.85 34.11,18.85 33.2,19.76 34.11,19.76 37.03,10.92 37.03,10.03 37.03,9.14 37.03,8.26 65.74,21.46 64.72,21.46 63.7,21.46 68.66,26.8 69.8,26.8 70.94,26.8 66.37,6.6 67.39,6.6 68.4,6.6 57.35,11.94 57.35,11.18 57.35,10.41 54.56,14.22 53.67,14.22 52.78,14.22 29.54,30.48 30.68,30.48 31.83,30.48 32.84,26.29 32.84,27.43 32.84,28.57 36.53,23.37 36.53,22.48 36.53,21.59 42.62,15.11 43.51,15.11 44.4,15.11 36.4,14.48 36.4,15.37 36.4,16.26 55.07,18.03 55.83,17.27 56.59,16.51 41.61,20.32 41.61,19.3 41.61,18.29 46.3,31.62 46.3,30.48 46.18,8.51
  pour Bottom (isolate 0.356): 18.67,33.53 18.67,-0.38 73.53,-0.38 73.53,33.53
  pour Top (isolate 0.356): -0.38,33.53 -0.38,-0.38 73.53,-0.38 73.53,33.53
GND*  (via drill 0.56)
  Top 0.508: C11.C v6.93,37.26 C11.C | JP1.1 4.52,36.63 C11.C | AMS1117-3.3.1 12.04,40.28 v12.01,40.31 | C12.C 6.93,40.31 v6.93,40.44
  Bottom 0.508: v12.01,40.31 7.19,40.31 | 7.19,40.31 6.93,40.06 v6.93,37.26 | v6.93,40.44 6.93,40.56 7.19,40.31
N$1  (via drill 0.41)
  other vias: 11.38,27.56 12.65,27.56 13.92,27.56 15.19,27.56 16.46,27.56 15.82,26.29 14.55,26.29 13.28,26.29 12.01,26.29 11.38,25.02 12.65,25.02 13.92,25.02 15.19,25.02 16.46,25.02 15.82,23.75 14.55,23.75 13.28,23.75 12.01,23.75
  pour Top: 0.76,26.67 6.73,26.67 11.18,22.23 19.18,22.23 19.18,28.83 arc-90 17.91,30.1 17.91,32.38 0.76,32.38
  pour Bottom: 23.24,22.23 11.18,22.23 6.73,26.67 0.76,26.67 0.76,32.38 17.91,32.38 17.91,30.1 arc90 19.18,28.83 23.24,28.83
N$2
  Top 0.254: Q2.G 32.52,23.12 32.13,22.73 32.13,13.59 32.38,13.34 37.72,13.34 38.86,14.48 41.13,14.48 41.78,13.82 | RR3.4 41.78,13.82 | 41.78,13.82 RR2.5
N$3  (via drill 0.41)
  other vias: 24.66,27.61 25.93,27.61 27.2,27.61 28.47,27.61 29.74,27.61 29.11,26.34 29.74,25.07 29.11,23.8 28.47,25.07 27.2,25.07 25.93,25.07 24.66,25.07 25.3,26.34 26.57,26.34 27.84,26.34 27.84,23.8 26.57,23.8 25.3,23.8
  pour Top: 0.76,22.23 5.97,22.23 11.81,16.38 31.24,16.38 31.24,28.32 23.88,28.32 23.88,21.59 10.79,21.59 6.35,26.04 0.76,26.04
  pour Bottom: 31.24,16.38 11.81,16.38 5.97,22.23 0.76,22.23 0.76,26.04 6.35,26.04 10.79,21.59 23.88,21.59 23.88,28.83 31.24,28.83
N$4
  Top 0.254: Q3.G 32.38,4.07 32.13,4.32 32.13,11.56 32.38,11.81 37.78,11.81 38.86,10.73 41.09,10.73 41.78,11.42 | RR3.1 41.78,11.42 | 41.78,11.42 RR2.8
N$5  (via drill 0.41)
  other vias: 24.69,8.56 25.96,8.56 27.23,8.56 28.5,8.56 29.77,8.56 29.13,7.29 29.77,6.02 28.5,6.02 27.23,6.02 25.96,6.02 24.69,6.02 25.32,7.29 26.59,7.29 27.86,7.29
  pour Top: 0.76,21.59 5.59,21.59 11.56,15.75 31.24,15.75 31.24,3.3 24,3.3 24,10.92 11.81,10.92 5.59,17.14 0.76,17.14
  pour Bottom: 31.24,5.46 23.88,5.46 23.88,10.92 11.81,10.92 5.71,17.02 0.76,17.02 0.76,21.59 5.59,21.59 11.43,15.75 31.24,15.75
N$6  (via drill 0.3)
  Top 0.254: Q1.G 23.12,23.12 23.5,23.5 23.5,28.19 24,28.7 31.37,28.7 31.62,28.45 31.62,13.21 32,12.83 38.92,12.83 v39.12,13.02 | RR2.6 RR3.3 v41.91,13.02
  Bottom 0.254: v39.12,13.02 v41.91,13.02
N$7  (via drill 0.3)
  Top 0.254: Q4.G 21.23,3.91 21.97,3.17 31.37,3.17 31.62,3.43 31.62,11.94 32,12.32 38.99,12.32 v39.12,12.19 | RR2.7 RR3.2 41.18,12.19 v41.91,12.19
  Bottom 0.254: v39.12,12.19 v41.91,12.19
N$8  (via drill 0.41)
  other vias: 11.33,8.56 12.6,8.56 13.87,8.56 15.14,8.56 16.41,8.56 15.77,7.29 16.41,6.02 15.14,6.02 13.87,6.02 12.6,6.02 11.33,6.02 11.96,7.29 13.23,7.29 14.5,7.29
  pour Bottom: 5.33,16.38 0.76,16.38 0.76,10.79 5.46,10.79 10.79,5.46 23.24,5.46 23.24,10.29 11.56,10.29
  pour Top: 17.78,0.64 5.71,0.64 5.71,8.89 arc90 3.81,10.92 0.89,10.92 0.89,16.26 5.33,16.26 11.43,10.16 17.78,10.16
N$9
  Top 0.254: R12.1 70.16,12.81 L1.A
N$10
  Top 0.254: U4.7 49.45,9.09 48.26,10.29 46.99,10.29 46.48,10.79 46.48,12.06 45.52,13.02 RR2.3
N$11
  Top 0.254: U4.5 51.99,9.35 51.82,9.53 49.78,9.53 48.51,10.79 47.24,10.79 46.99,11.05 46.99,12.32 45.48,13.82 RR2.4
N$12
  Top 0.254: RR2.1 45.22,11.42 45.47,11.18 45.47,11.05 45.21,10.79 43.05,10.79 41.78,9.53 40.01,9.53 39.8,9.32 U5.7
N$13
  Top 0.254: U5.5 42.34,9.32 43.31,10.29 45.47,10.29 45.97,10.79 45.97,11.81 45.56,12.22 RR2.2
N$29
  Top 0.254: Y1.1 50.84,17.36 49.4,18.8 49.15,18.8 48.28,19.67 U1.7
N$30
  Top 0.254: Y1.3 49.47,19.36 49.28,19.56 49.15,19.68 49.08,19.75 U1.8
N$33
  Top 0.254: U1.20 46.68,29.53 48.07,30.92 C3.2
RESET  (via drill 0.3)
  Top 0.254: JST1.4 66.72,20.74 66.55,20.57 66.55,20.07 66.04,19.56 61.21,19.56 59.05,21.72 59.05,22.48 58.8,22.73 v56.77,22.73 56.52,22.73 53.72,25.53 53.72,26.67 52.13,28.26 R4.1 | U1.29 44.09,24.24 v44.2,24.26
  Bottom 0.254: v56.77,22.73 56.13,22.73 53.85,25.02 45.21,25.02 44.45,24.26 v44.2,24.26
VCC  (via drill 0.56)
  Top 0.508: C2.2 44.45,2.45 v44.32,2.41 | C10.2 54.01,4.66 v54.36,4.32
  Bottom 0.508: J4.VIN 34.51,12.23 35.18,11.56 35.18,3.94
  pour Bottom (no thermals): 73.03,0 4.45,0 arc160 0.64,4.95 0.64,10.16 5.08,10.16 10.79,4.57 72.39,4.57

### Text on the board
tPlace: W | B | G | R | V1.0 | 2018/03 | VCC | GND | VCC | LED RGBW CONTROLLER
bPlace: +5V | +3V3 | GND | POWER SUPPLY | 5V TO 3.3V | +5V | +3V3 | GND | POWER SUPPLY | 24V TO 5V | MAX 24V

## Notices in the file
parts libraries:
SparkFun-DigitalIC: Licensing: Creative Commons ShareAlike 4.0 International - https://creativecommons.org/licenses/by-sa/4.0
